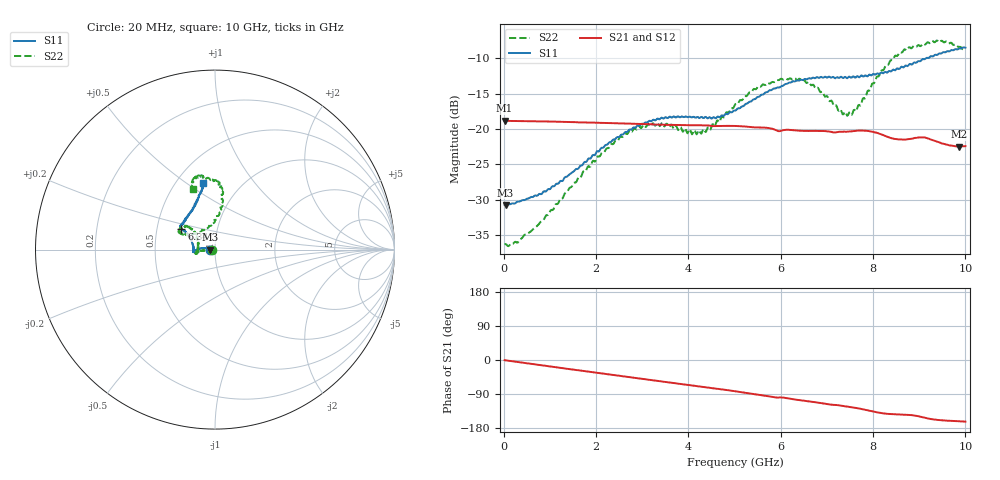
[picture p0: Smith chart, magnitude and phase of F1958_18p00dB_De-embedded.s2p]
! Integrated Device Technology
! Corporate Headquarters
! 6024 Silver Creek Valley Road
! San Jose, CA 95138  USA
! Phone:  1-408-284-8200
! Toll Free:  1-800-223-1366
! Webpage:  http://www.idt.com/
! Timing and RF Division
! 515 Groton Road, Suite 102
! Westford, MA 01886-6024
! Device:  F1958
! Description: 7-bit 0.25 dB Digital Step Attenuator
! Frequency:  0.001 -  6.000 GHz
! Package:  4x4 mm Thin QFN Plastic Package: 24 pin
! Ports:  2 RF, 12 DC
!  Pin  1  = D0
!  Pin  2  = VDD
!  Pin  3  = VMODE
!  Pin  4  = GND
!  Pin  5  = RF1  =  Port 1
!  Pin  6  = GND
!  Pin  7  = GND
!  Pin  8  = GND
!  Pin  9  = GND
!  Pin 10  = GND
!  Pin 11  = GND
!  Pin 12  = GND
!  Pin 13  = GND
!  Pin 14  = RF2  =  Port 2
!  Pin 15  = GND
!  Pin 16  = LE
!  Pin 17  = CLK
!  Pin 18  = DATA
!  Pin 19  = D6
!  Pin 20  = D5
!  Pin 21  = D4
!  Pin 22  = D3
!  Pin 23  = D2
!  Pin 24  = D1
! State:  72
! Atten State:  18.00 dB
! Voltage:  +3.30 Volts
! Current:  0.258 mA
! Data:  The device was measured on a F1958 evaluation board which has
!  individual transmission lines to the RF pins.  Data was collected
!  using a calibrated network analyzer.  The evaluation board was
!  de-embedded using Automatic Fixture Removal (AFR).
!  The reference plane is the edge of the package pin.
! Misc:
!  Action Tracker AT0419
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# GHz S dB R 50
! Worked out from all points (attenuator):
!   500 points, 20 MHz to 10 GHz, reference 50 ohm
!   highest |S21| = -18.82 dB at 20 MHz (marker M1); lowest = -22.5 dB at 9.86 GHz (marker M2)
!   lowest |S11| = -30.7 dB at 40 MHz (marker M3), VSWR 1.06, Z = 47.2 - j0.0464 ohm
!   |S11| at or under -10 dB: start of sweep to 9.139 GHz
!   |S22| runs from -36.6 to -7.5 dB; largest |S21 - S12| = 0.00041
!   S11 on the Smith chart (normalised r, x): 20 MHz: 0.94, -0.00; 6.34 GHz: 0.67, +0.16; 10 GHz: 0.68, +0.58
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0.02  -30.70 -178.9  -18.82 -0.4  -18.82 -0.4  -36.31 -177.0
0.04  -30.74 -179.0  -18.83 -0.8  -18.82 -0.8  -36.24 -175.6
0.32  -30.24 175.3  -18.86 -5.5  -18.86 -5.5  -35.92 -179.3
0.72  -29.43 173.2  -18.89 -12.2  -18.89 -12.2  -33.71 -176.0
1.7  -25.12 172.3  -19.04 -28.4  -19.03 -28.4  -26.34 -176.8
2.6  -20.67 178.3  -19.21 -43.2  -19.19 -43.2  -20.86 -173.6
2.92  -19.49 -178.0  -19.26 -48.4  -19.24 -48.5  -19.61 -170.7
3.36  -18.59 -174.5  -19.36 -55.7  -19.36 -55.8  -19.41 -166.7
4.3  -18.31 -178.7  -19.45 -70.8  -19.47 -70.8  -20.35 164.4
4.64  -18.20 172.8  -19.56 -76.1  -19.57 -76.2  -18.78 151.5
5.02  -17.37 161.6  -19.55 -82.6  -19.56 -82.7  -16.45 139.9
5.56  -15.25 151.0  -19.77 -92.1  -19.78 -92.1  -14.01 140.3
6.34  -13.14 148.1  -20.18 -104.8  -20.20 -104.8  -13.01 153.6
6.68  -12.77 146.8  -20.25 -110.1  -20.26 -110.0  -13.77 153.8
7.3  -12.59 141.0  -20.36 -120.4  -20.37 -120.3  -17.22 132.5
7.5  -12.62 138.3  -20.33 -123.8  -20.33 -123.7  -17.61 113.7
7.68  -12.58 135.4  -20.21 -127.5  -20.20 -127.5  -16.61 96.3
8.34  -11.80 119.3  -21.15 -142.3  -21.15 -142.4  -10.77 81.1
8.68  -11.15 112.5  -21.49 -144.2  -21.48 -144.2  -8.70 85.9
9.26  -9.67 104.7  -21.49 -155.9  -21.49 -156.0  -7.63 99.2
9.86  -8.61 99.8  -22.47 -161.4  -22.50 -161.3  -8.38 108.7
10  -8.48 99.8  -22.41 -162.6  -22.44 -162.4  -8.92 109.7
